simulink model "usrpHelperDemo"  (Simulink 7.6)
settings: Solver=FixedStepDiscrete  StartTime=0.0  StopTime=inf  RelTol=1e-3
PostLoadFcn:
  | set_param([gcs,'/usrp_helper'],'firmware','');
  | set_param([gcs,'/usrp_helper'],'bitstream','')
undefined symbols (not defined in the file or in its folder): array, Bit, Channels, Complex, Concatenate, D, Demo, frames, Fs, get, INT16, kB, kSps, Mbit, N, S, s, usrp_helper
libraries: usrp_GPP x4, dspsnks4 x4, simulink x2

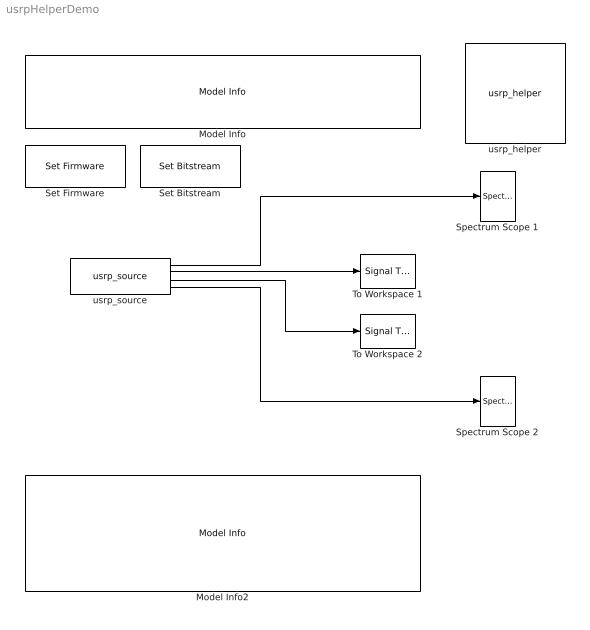
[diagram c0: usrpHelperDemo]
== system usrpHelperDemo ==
  Model Info : simulink/Model-Wide Utilities/Model Info  SystemSampleTime=-1  InitialBlockCM=None  BlockCM=None  Frame=on  DisplayStringWithTags=usrp_helper Demo  HorizontalTextAlignment=Center  LeftAlignmentValue=0.5  SourceBlockDiagram=usrpHelperDemo  TagMaxNumber=20
  Model Info2 : simulink/Model-Wide Utilities/Model Info  SystemSampleTime=-1  InitialBlockCM=None  BlockCM=None  Frame=on  DisplayStringWithTags=|  HorizontalTextAlignment=Center  LeftAlignmentValue=0.5  SourceBlockDiagram=usrpHelperDemo  TagMaxNumber=20
      | This model configures the USRP to be able to
      | receive four data streams at once. This is
      | done by using the usrp_helper block to select
      | a non-standard FPGA bitstream file.
      | 
      | Since only BasicRX and LFRX daughterboards
      | offer two subdevices, you need either of these
      | boards to run this demo.
  Set Bitstream : usrp_GPP/Set Bitstream  SystemSampleTime=-1  bitfile=zwei.rbf
  Set Firmware : usrp_GPP/Set Firmware  SystemSampleTime=-1  bitfile=zwei.rbf
  Spectrum Scope 1 : dspsnks4/Spectrum Scope  DialogController=dspdialog.SpectrumScope  DialogControllerArgs=DataTag0  SystemSampleTime=-1  ScopeProperties=on  Domain=Frequency  HorizSpan=1  UseBuffer=off  BufferSize=128  Overlap=64  inpFftLenInherit=off  FFTlength=128  numAvg=2  DisplayProperties=off  AxisGrid=on  Memory=off  FrameNumber=on  AxisLegend=off  AxisZoom=off  OpenScopeAtSimStart=on  OpenScopeImmediately=off  FigPos=get(0,'defaultfigureposition')  AxisProperties=off  XUnits=Hertz  XRange=[-Fs/2...Fs/2]  XDisplay=0  InheritXIncr=on  XIncr=1.0  XLabel=Samples  XLimit=Auto  YUnits=dB  XMax=1  XMin=0  YLabel=Magnitude-squared, dB  LineProperties=off  wintypeSpecScope=Hann  RsSpecScope=50  betaSpecScope=5  winsampSpecScope=Periodic  XAxisParamsVer=6.8
  Spectrum Scope 2 : dspsnks4/Spectrum Scope  DialogController=dspdialog.SpectrumScope  DialogControllerArgs=DataTag1  SystemSampleTime=-1  ScopeProperties=on  Domain=Frequency  HorizSpan=1  UseBuffer=off  BufferSize=128  Overlap=64  inpFftLenInherit=off  FFTlength=128  numAvg=2  DisplayProperties=off  AxisGrid=on  Memory=off  FrameNumber=on  AxisLegend=off  AxisZoom=off  OpenScopeAtSimStart=on  OpenScopeImmediately=off  FigPos=get(0,'defaultfigureposition')  AxisProperties=off  XUnits=Hertz  XRange=[-Fs/2...Fs/2]  XDisplay=0  InheritXIncr=on  XIncr=1.0  XLabel=Samples  XLimit=Auto  YUnits=dB  XMax=1  XMin=0  YLabel=Magnitude-squared, dB  LineProperties=off  wintypeSpecScope=Hann  RsSpecScope=50  betaSpecScope=5  winsampSpecScope=Periodic  XAxisParamsVer=6.8
  To Workspace 1 : dspsnks4/Signal To Workspace  SystemSampleTime=-1  VariableName=yout1  FrameMode=Concatenate frames (2-D array)
  To Workspace 2 : dspsnks4/Signal To Workspace  SystemSampleTime=-1  VariableName=yout2  FrameMode=Concatenate frames (2-D array)
  usrp_helper : usrp_GPP/usrp_helper  usrp_number=0  serial_number=S/N: .  daughterboards_rx=RX A: Flex 2400 Rx, RX B: Flex 2400 Rx,  daughterboards_tx=TX A: Flex 2400 Tx, TX B: Flex 2400 Tx.  usb_block_size=0  usb_nblocks=0  firmware=Please include USB firmware!  bitstream=C:\MATLAB\R2009b\simulink-usrp_2.1.0\firmware\rev4\std_4rx_0tx.rbf  sample_time_factor=1
  usrp_source : usrp_GPP/usrp_source  usrp_number=0  serial_number=Unknown (USRP Board #0 not found).  decimation=256  sample_width=16 Bit  sampling_rate_and_bandwidth=4 Channels: 1000 kSps, 3906.25 kB/s, 30.5176 Mbit/s.  vector_length=1024  sideA_subdev1_tab_=0  sideA_subdev1_subdevice=Unknown (USRP Board #0 not found).  sideA_subdev1_datatype=INT16 Complex  sideA_subdev1_frequency_range=Unknown.  sideA_subdev1_frequency_port=off  sideA_subdev1_frequency=30e6  sideA_subdev1_gain_range=Unknown.  sideA_subdev1_gain=0  sideA_subdev1_antenna=Not applicable  sideA_subdev2_tab_=0  sideA_subdev2_subdevice=Unknown (USRP Board #0 not found).  sideA_subdev2_datatype=INT16 Complex  sideA_subdev2_frequency_range=Unknown.  sideA_subdev2_frequency_port=off  sideA_subdev2_frequency=30e6  sideA_subdev2_gain_range=Unknown.  sideA_subdev2_gain=0  sideB_subdev1_tab_=0  sideB_subdev1_subdevice=Unknown (USRP Board #0 not found).  sideB_subdev1_datatype=INT16 Complex  sideB_subdev1_frequency_range=Unknown.  sideB_subdev1_frequency_port=off  sideB_subdev1_frequency=30e6  sideB_subdev1_gain_range=Unknown.  sideB_subdev1_gain=0  sideB_subdev1_antenna=Not applicable  sideB_subdev2_subdevice=Unknown (USRP Board #0 not found).  sideB_subdev2_datatype=INT16 Complex  sideB_subdev2_frequency_range=Unknown.  sideB_subdev2_frequency_port=off  sideB_subdev2_frequency=30e6  sideB_subdev2_gain_range=Unknown.  sideB_subdev2_gain=0
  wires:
  usrp_source/1 -> Spectrum Scope 1/1
  usrp_source/3 -> To Workspace 2/1
  usrp_source/4 -> Spectrum Scope 2/1
  usrp_source/2 -> To Workspace 1/1
